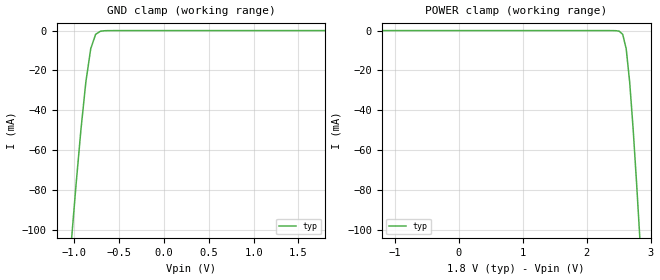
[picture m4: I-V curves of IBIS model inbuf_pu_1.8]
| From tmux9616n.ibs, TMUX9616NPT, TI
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| inbuf_pu_1.8
[Model]   inbuf_pu_1.8
Model_type   Input
Vinl = 0.54
Vinh = 1.08
|   typ   min   max
C_comp   1.008417e-12   NA   NA
[Voltage Range]   1.8   NA   NA
[Temperature Range]   27   NA   NA
[Power Clamp Reference]   1.8   NA   NA
[GND Clamp Reference]   0   NA   NA
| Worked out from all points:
|   GND clamp passes 1 mA (typ) near -0.73 V on its own axis
[GND Clamp]
|   Voltage   I(typ)   I(min)   I(max)
-3.6V     -1.746A    NA         NA
-1.036V   -107mA     NA         NA
-981.8mV  -77.23mA   NA         NA
-927.3mV  -49.65mA   NA         NA
-872.7mV  -25.85mA   NA         NA
-818.2mV  -9.103mA   NA         NA
-763.6mV  -1.887mA   NA         NA
-709.1mV  -296.2uA   NA         NA
-654.5mV  -59.49uA   NA         NA
1.8V      13.02pA    NA         NA
[POWER Clamp]
|   Voltage   I(typ)   I(min)   I(max)
-1.8V     37.73pA    NA         NA
2.509V    -296.2uA   NA         NA
2.564V    -1.887mA   NA         NA
2.618V    -9.103mA   NA         NA
2.673V    -25.85mA   NA         NA
2.727V    -49.65mA   NA         NA
2.782V    -77.23mA   NA         NA
2.836V    -107mA     NA         NA
3.6V      -577.7mA   NA         NA
